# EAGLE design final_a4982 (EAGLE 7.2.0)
CNAME: A4982 STEPPER MOTOR DRIVER; CREVISION: 1.0; DESIGNER: RODNEYD
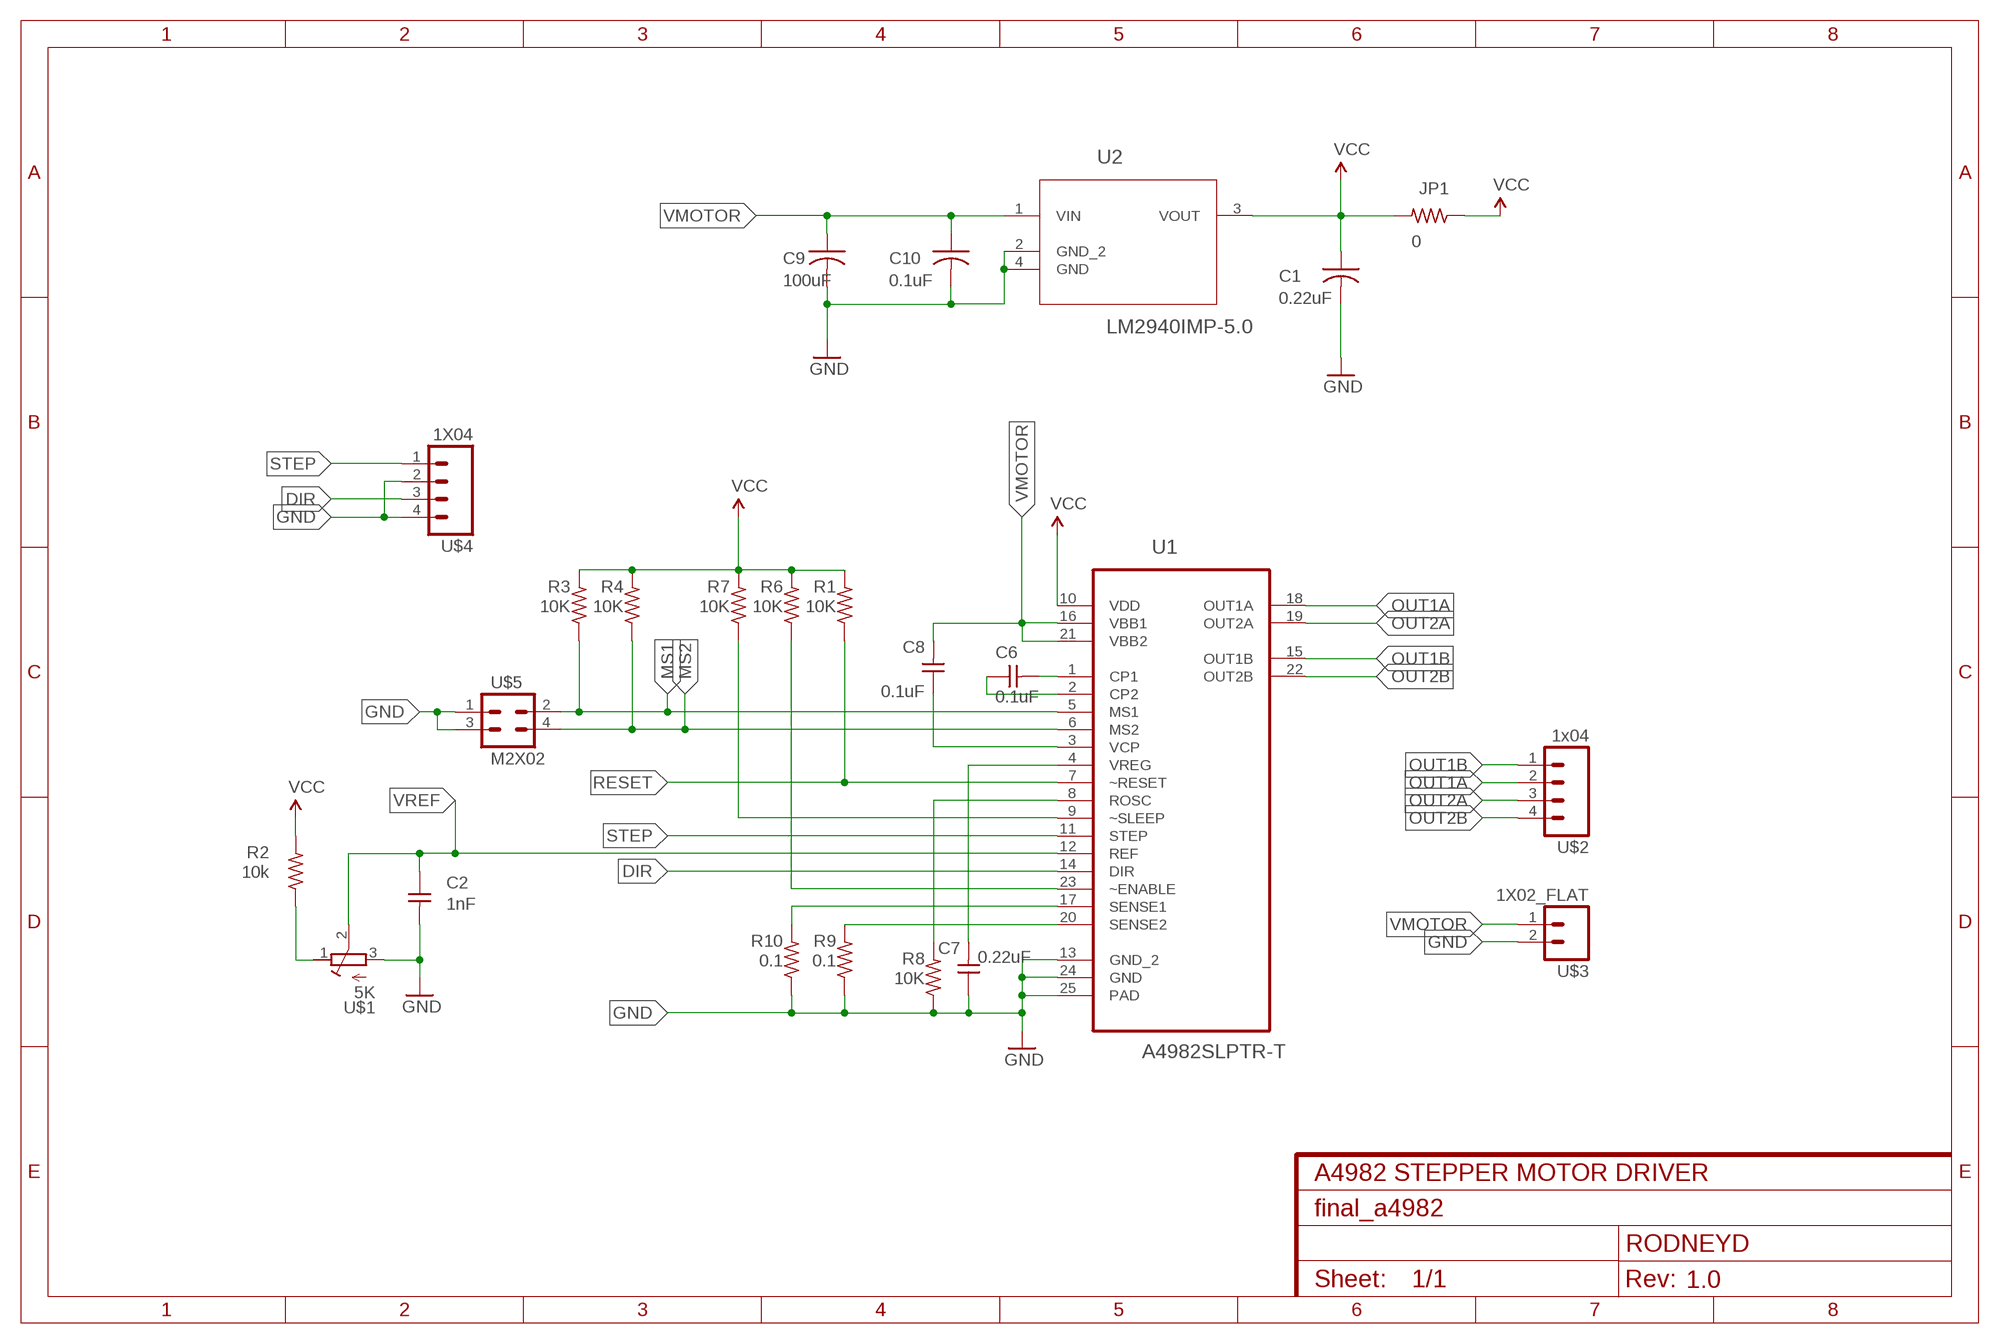
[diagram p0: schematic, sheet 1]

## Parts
C1  0.22uF  CAP-POLARIZED1206FAB  [C1206FAB]
C2  1nF  CAPFAB  [C1206FAB]
C6  0.1uF  CAPFAB  [C1206FAB]
C7  0.22uF  CAPFAB  [C1206FAB]
C8  0.1uF  CAPFAB  [C1206FAB]
C9  100uF  CAP-POLARIZED6.3MM_ELECTROLYTIC  [CAPAE660X610N]
C10  0.1uF  CAP-POLARIZED1206FAB  [C1206FAB]
JP1  0  RESISTOR1206FAB  [R1206FAB]
R1  10K  RESISTOR1206FAB  [R1206FAB]
R2  10k  RESISTOR1206FAB  [R1206FAB]
R3  10K  RESISTOR1206FAB  [R1206FAB]
R4  10K  RESISTOR1206FAB  [R1206FAB]
R6  10K  RESISTOR1206FAB  [R1206FAB]
R7  10K  RESISTOR1206FAB  [R1206FAB]
R8  10K  RESISTOR1206FAB  [R1206FAB]
R9  0.1  RESISTOR1210  [R1210]
R10  0.1  RESISTOR1210  [R1210]
U1  A4982SLPTR-T  [SOP65P640X120-25N]
U2  LM2940IMP-5.0  [SOT230P696X180-4N]
U$1  5K  POTENTIOMETER  [TC33X]
U$2  1x04  M041X04_SMD_STRAIGHT_ALT  [1X04_SMD_STRAIGHT_ALT]
U$3  1X02_FLAT  M02  [1X02_SMD_FLAT_PADS]
U$4  1X04  M041X04_SMD_STRAIGHT_ALT  [1X04_SMD_STRAIGHT_ALT]
U$5  M2X02  [2X2_SMD]

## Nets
DIR: U1.14(DIR) U$4.3
GND: C1.2 C2.2 C7.1 C9.2 C10.2 R8.1 R9.1 R10.1 U1.13(GND_2) U1.24(GND) U1.25(PAD) U2.2(GND_2) U2.4(GND) U$1.3(E) U$3.2 U$4.2 U$4.4 U$5.1 U$5.3
MS1: R3.1 U1.5(MS1) U$5.2
MS2: R4.1 U1.6(MS2) U$5.4
N$1: C6.2 U1.1(CP1)
N$2: R7.1 U1.9(~SLEEP)
N$5: R6.1 U1.23(~ENABLE)
N$6: C6.1 U1.2(CP2)
N$9: C7.2 U1.4(VREG)
N$10: C8.1 U1.3(VCP)
N$20: R8.2 U1.8(ROSC)
N$22: R10.2 U1.17(SENSE1)
N$23: R9.2 U1.20(SENSE2)
OUT1A: U1.18(OUT1A) U$2.2
OUT1B: U1.15(OUT1B) U$2.1
OUT2A: U1.19(OUT2A) U$2.3
OUT2B: U1.22(OUT2B) U$2.4
POT1: R2.1 U$1.1(A)
RESET: R1.1 U1.7(~RESET)
STEP: U1.11(STEP) U$4.1
VCC: C1.1 JP1.1 JP1.2 R1.2 R2.2 R3.2 R4.2 R6.2 R7.2 U1.10(VDD) U2.3(VOUT)
VMOTOR: C8.2 C9.1 C10.1 U1.16(VBB1) U1.21(VBB2) U2.1(VIN) U$3.1
VREF: C2.1 U1.12(REF) U$1.2(S)

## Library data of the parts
C1 C9 C10 = Working:CAP-POLARIZED
C2 C6-C8 = Working:CAP
JP1 R1-R4 R6-R10 = Working:RESISTOR: Resistor (US Symbol)
U1 = Working:A4982SLPTR-T: DMOS Microstepping Driver with Translator and Overcurrent Protection; MPN: A4982SLPTR-T; OC_FARNELL: -; OC_NEWARK: 67R9668; PACKAGE: TSSOP-24; SUPPLIER: Allegro
U2 = Working:LM2940IMP-5.0: Low Dropout Regulator; MPN: LM2940IMP-50; OC_FARNELL: 9778845; OC_NEWARK: 41K4582; PACKAGE: SOT-223-4; SUPPLIER: National
U$1 = Working:POTENTIOMETER
U$2 U$4 = Working:M04
U$3 = Working:M02
U$5 = Working:M2X02

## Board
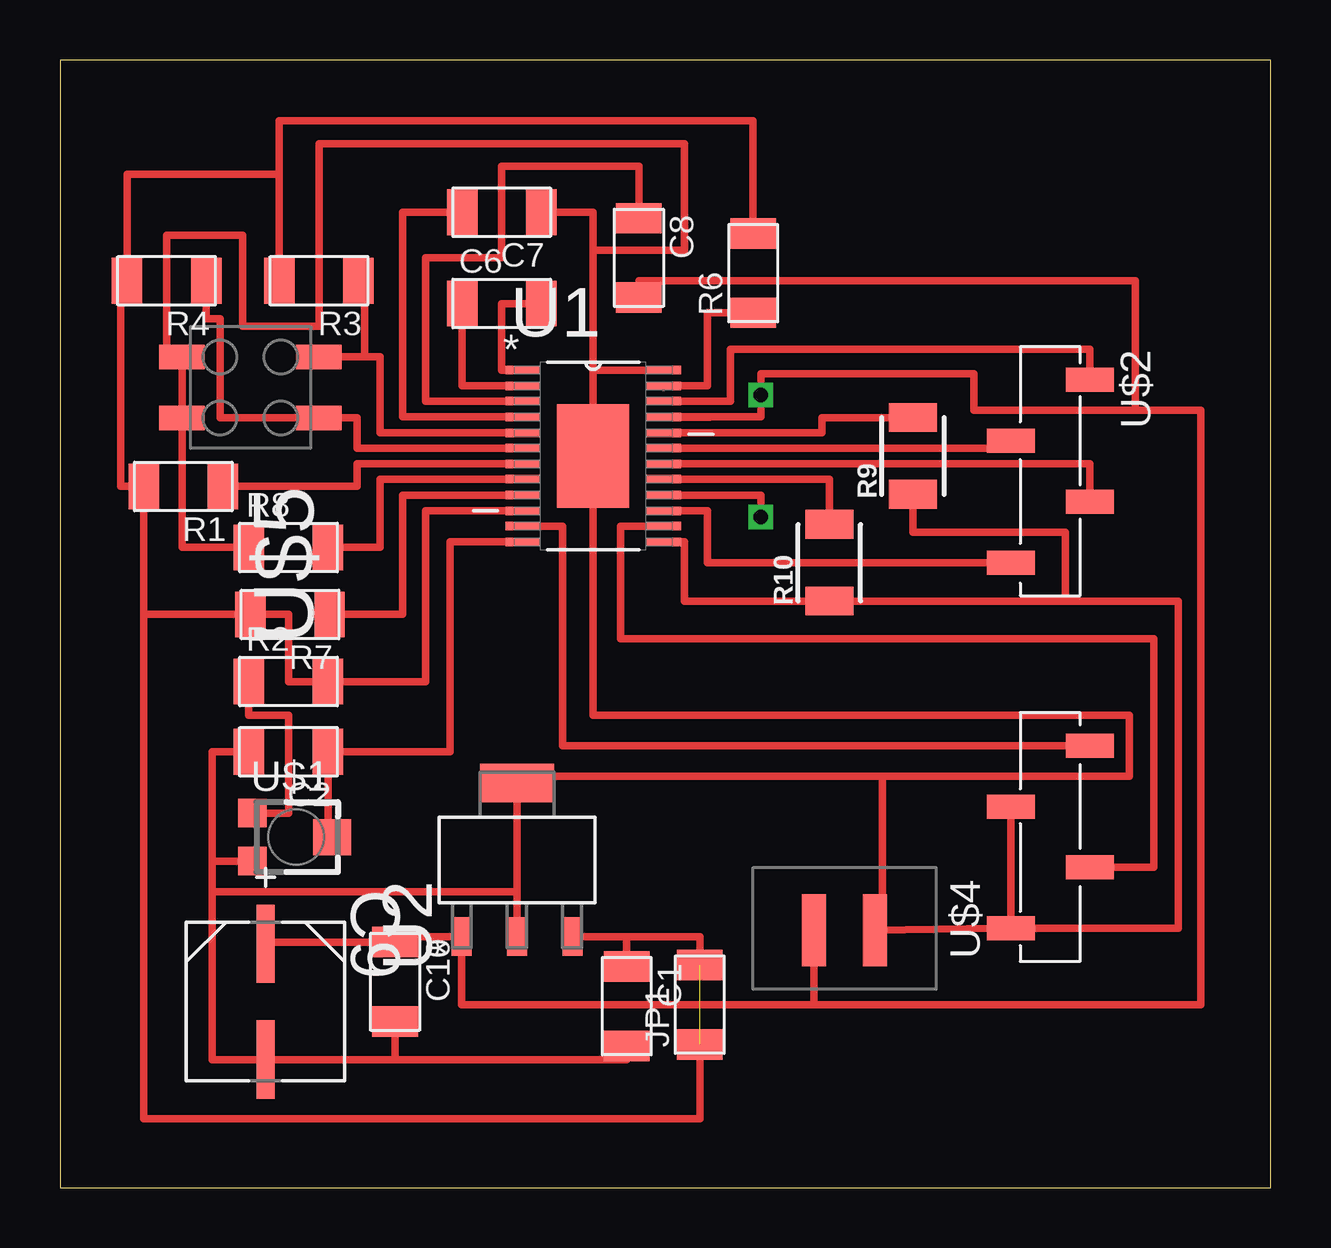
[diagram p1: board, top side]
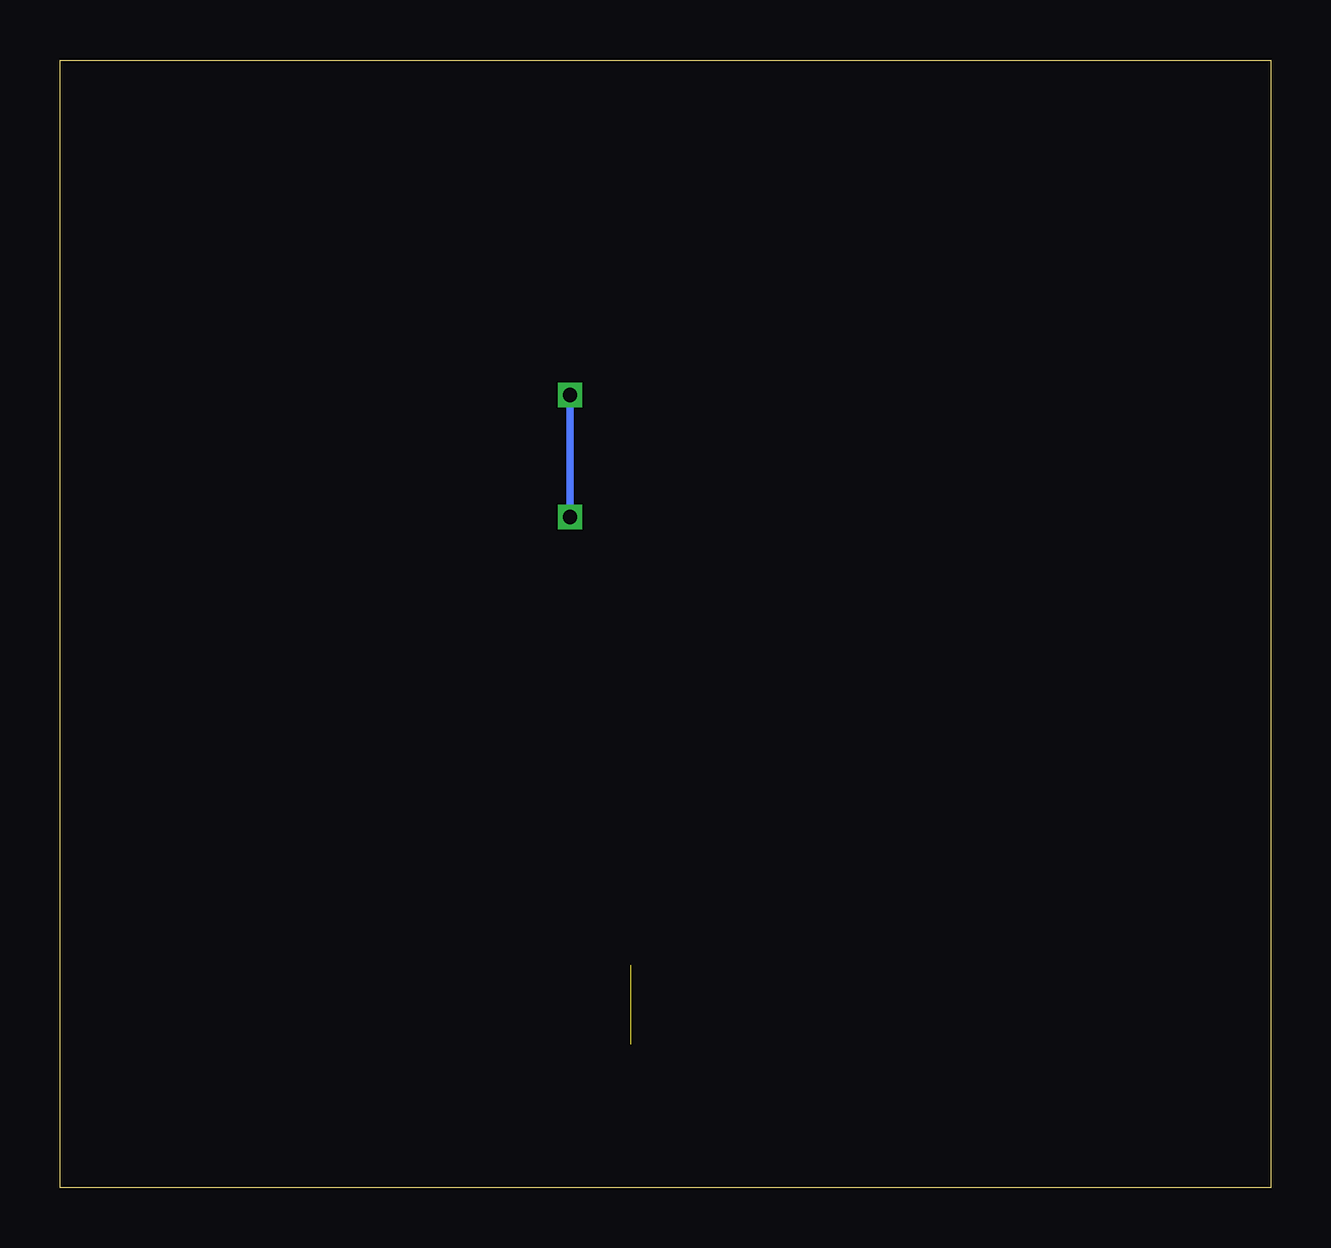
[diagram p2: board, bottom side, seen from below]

Size 50.47 x 46.98 mm. Coordinates in mm from the lower left corner, seen from the top.
Outline: 0,0 50.47,0 50.47,46.98 0,46.98 0,0
Copper layers (1*16): Top 0.035mm / dielectric 1.5mm / Bottom 0.035mm
Design rules "default *": minimum track width 12mil, minimum drill 24mil, track to track 12mil, track to pad 12mil, pad to pad 8mil, via to via 8mil, smd to smd 8mil, copper to edge 20mil, drill to drill 8mil, minimum pad ring 10mil, minimum via ring 8mil, stop-mask expansion 4mil, vias tented up to drill 0mil, thermal gap 10mil

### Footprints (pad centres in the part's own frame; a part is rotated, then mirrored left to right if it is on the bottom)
C1206FAB = smd 1.27 x 1.905: 1 -1.651,0; 2 1.651,0
CAPAE660X610N = smd 3.251 x 0.762: 1 2.667,0; 2 7.493,0
R1206FAB = smd 1.27 x 1.905: 1 -1.651,0; 2 1.651,0
R1210 = smd 1.2 x 2: 1 -1.6,0; 2 1.6,0
SOP65P640X120-25N = smd 1.473 x 0.356: 1 -2.921,3.581; 2 -2.921,2.921; 3 -2.921,2.286; 4 -2.921,1.626; 5 -2.921,0.965; 6 -2.921,0.33; 7 -2.921,-0.33; 8 -2.921,-0.965; 9 -2.921,-1.626; 10 -2.921,-2.286; 11 -2.921,-2.921; 12 -2.921,-3.581; 13 2.921,-3.581; 14 2.921,-2.921; 15 2.921,-2.286; 16 2.921,-1.626; 17 2.921,-0.965; 18 2.921,-0.33; 19 2.921,0.33; 20 2.921,0.965; 21 2.921,1.626; 22 2.921,2.286; 23 2.921,2.921; 24 2.921,3.581 | smd 2.997 x 4.318: 25 0,0
SOT230P696X180-4N = smd 1.6 x 0.838: 1 -3.2,2.311; 2 -3.2,0; 3 -3.2,-2.311 | smd 1.6 x 3.099: 4 3.2,0
TC33X = smd 1.2 x 1.2: 1 -1,-1.825; 3 1,-1.825 | smd 1.5 x 1.6: 2 0,1.5
1X04_SMD_STRAIGHT_ALT = smd 1 x 2: 1 -1.27,-0.38; 2 -3.81,2.92; 3 -6.35,-0.38; 4 -8.89,2.92
1X02_SMD_FLAT_PADS = smd 1 x 3: 1 2.54,1.19; 2 5.08,1.19
2X2_SMD = smd 1.02 x 1.9: 1 1.27,-0.31; 2 1.27,5.39; 3 3.81,-0.31; 4 3.81,5.39

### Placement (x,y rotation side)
C1  23.62,7.56 270 top
C2  9.53,18.16 180 top
C6  18.41,36.83 0 top
C7  18.41,40.64 180 top
C8  24.13,38.73 270 top
C9  8.57,12.83 270 top
C10  13.97,8.57 270 top
JP1  26.67,7.62 90 top
R1  5.14,29.21 180 top
R2  9.53,21.08 0 top
R3  10.79,37.78 180 top
R4  4.45,37.78 180 top
R6  28.89,38.1 90 top
R7  9.59,23.88 180 top
R8  9.53,26.67 0 top
R9  35.56,30.48 90 top
R10  32.07,26.04 90 top
U1  22.23,30.48 0 top
U2  19.05,13.65 90 top
U$1  9.84,14.61 270 top
U$2  40.01,24.77 270 top
U$3  28.89,9.53 0 top
U$4  42.55,19.68 90 top
U$5  5.4,35.88 270 top

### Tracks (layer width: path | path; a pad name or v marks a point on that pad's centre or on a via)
DIR
  Top 0.305: U1.14 23.37,27.56 23.37,22.86 45.59,22.86 45.59,13.34 U$4.3
GND
  Top 0.305: 22.23,34.06 U1.25 22.23,19.68 44.58,19.68 44.58,17.14 34.29,17.14 | 22.23,34.06 U1.24 | U1.13 26.04,26.9 26.04,24.43 R10.1 41.91,24.43 | 22.23,34.06 22.23,39.05 | 22.23,39.05 22.23,40.64 C7.1 | 33.97,10.79 U$3.2 | U$3.2 39.05,10.79 U$4.4 | U2.2 19.05,12.32 | 19.05,12.32 U2.4 20.32,17.14 34.29,17.14 | R8.1 5.09,26.67 U$5.3 U$5.1 4.45,34.61 4.45,39.69 7.62,39.69 7.62,35.88 10.79,35.88 10.79,43.5 26.04,43.5 26.04,39.05 22.23,39.05 | 6.35,12.32 19.05,12.32 | 6.35,12.32 6.35,5.33 C9.2 13.97,5.33 | R9.1 35.56,27.3 41.91,27.3 41.91,24.43 | 41.91,24.43 46.61,24.43 46.61,10.79 U$4.4 | C2.2 6.35,18.16 6.35,13.61 | 6.35,13.61 6.35,12.32 | U$4.2 U$4.4 | U$1.3 6.35,13.61 | 13.97,5.33 C10.2 | C1.2 23.62,5.33 13.97,5.33 | U$3.2 34.29,10.71 34.29,17.14
MS1
  Top 0.305: U$5.2 12.7,34.61 | 12.7,34.61 13.34,34.61 13.34,31.45 U1.5 | R3.1 12.7,37.78 12.7,34.61
MS2
  Top 0.305: U1.6 19.3,30.8 12.38,30.8 12.38,32.07 U$5.4 6.67,32.07 6.67,36.2 6.1,36.2 R4.1
N$1
  Top 0.305: U1.1 18.41,34.06 18.41,36.83 C6.2
N$2
  Top 0.305: U1.9 14.29,28.85 14.29,23.88 R7.1
N$5
  Top 0.305: 25.15,33.34 U1.23 26.99,33.4 26.99,36.45 R6.1
N$6
  Top 0.305: U1.2 16.76,33.4 C6.1
N$9
  Top 0.305: C7.2 14.29,40.64 14.29,32.11 U1.4
N$10
  Top 0.305: U1.3 15.24,32.77 15.24,38.73 18.41,38.73 18.41,42.55 24.13,42.55 C8.1
N$20
  Top 0.305: U1.8 13.34,29.52 13.34,26.67 R8.2
N$22
  Top 0.305: U1.17 32.07,29.52 R10.2
N$23
  Top 0.305: U1.20 31.75,31.45 31.75,32.08 R9.2
OUT1A
  Top 0.305: U1.18 42.92,30.15 U$2.2
OUT1B
  Top 0.305: U1.15 26.99,28.19 26.99,26.04 U$2.1
OUT2A
  Top 0.305: U1.19 39.62,30.81 U$2.3
OUT2B
  Top 0.305: U1.22 27.94,32.77 27.94,34.92 42.92,34.92 U$2.4
POT1
  Top 0.305: R2.1 7.87,19.68 9.53,19.68 9.53,15.61 U$1.1
RESET
  Top 0.305: U1.7 12.38,30.15 12.38,29.21 R1.1
STEP
  Top 0.305: U1.11 20.95,27.56 20.95,18.41 U$4.1
VCC  (1 unrouted)
  Top 0.305: R3.2 9.14,42.23 | 9.14,42.23 2.79,42.23 R4.2 2.54,37.78 2.54,29.21 R1.2 3.49,23.88 | 3.49,23.88 R7.2 9.53,23.88 9.53,21.08 R2.2 15.24,21.08 15.24,28.19 U1.10 | R6.2 28.89,44.45 9.14,44.45 9.14,42.23 | C1.1 23.62,10.45 | 23.62,10.45 U2.3 | 23.62,10.45 26.67,10.45 JP1.2 | JP1.1 26.67,2.86 3.49,2.86 3.49,23.88
VMOTOR  (via drill 0.6)
  Top 0.305: U1.21 29.21,32.11 | 29.21,32.11 25.08,32.07 | C9.1 8.57,10.22 C10.1 13.97,10.45 U2.1 16.74,7.62 31.43,7.62 | U1.16 29.21,28.85 v29.21,27.94 | 29.21,32.11 v29.21,33.02 29.21,33.91 38.1,33.91 38.1,32.38 44.83,32.38 | 44.83,32.38 44.83,37.78 24.13,37.78 C8.2 | 44.83,32.38 47.56,32.38 47.56,7.62 31.43,7.62 | 31.43,7.62 U$3.1
  Bottom 0.305: v29.21,27.94 v29.21,33.02
VREF
  Top 0.305: U1.12 16.26,26.9 16.26,18.16 C2.1 11.18,14.61 U$1.2

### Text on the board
tDocu: MOTOR | CTRL | VM | GND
